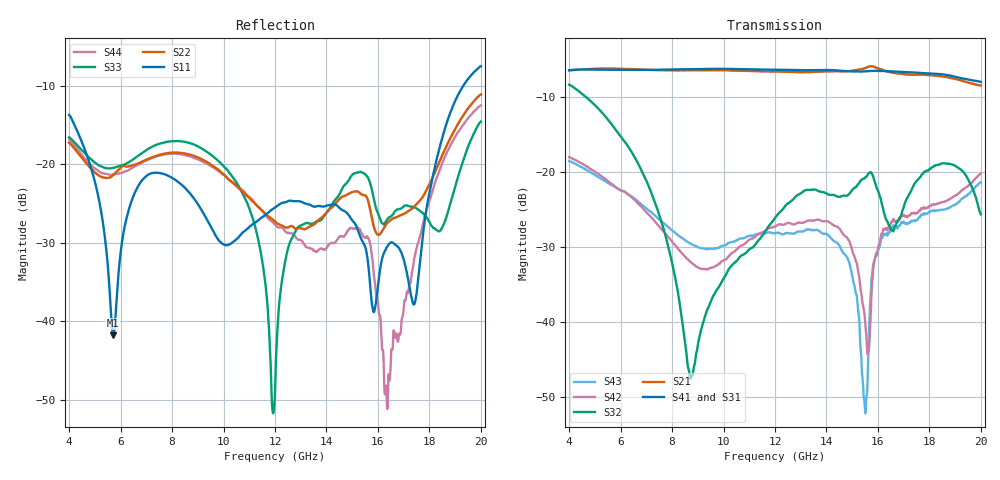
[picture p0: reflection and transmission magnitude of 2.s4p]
!Keysight Technologies,N5247B,US57180241,A.12.85.04
!Date: Friday, March 23, 2018 09:48:32
!Correction: S11(Full 4 Port(1,2,3,4))
!S12(Full 4 Port(1,2,3,4))
!S13(Full 4 Port(1,2,3,4))
!S14(Full 4 Port(1,2,3,4))
!S21(Full 4 Port(1,2,3,4))
!S22(Full 4 Port(1,2,3,4))
!S23(Full 4 Port(1,2,3,4))
!S24(Full 4 Port(1,2,3,4))
!S31(Full 4 Port(1,2,3,4))
!S32(Full 4 Port(1,2,3,4))
!S33(Full 4 Port(1,2,3,4))
!S34(Full 4 Port(1,2,3,4))
!S41(Full 4 Port(1,2,3,4))
!S42(Full 4 Port(1,2,3,4))
!S43(Full 4 Port(1,2,3,4))
!S44(Full 4 Port(1,2,3,4))
!S4P File: Measurements: <S11,S12,S13,S14>,
!<S21,S22,S23,S24>,
!<S31,S32,S33,S34>,
!<S41,S42,S43,S44>:
# Hz S  dB  R 50
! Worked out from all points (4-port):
!   6401 points, 4 GHz to 20 GHz, reference 50 ohm
!   strongest paths, dB at 4 GHz, 8 GHz, 12 GHz, 16 GHz, 20 GHz:
!     S41: -6.4, -6.3, -6.3, -6.5, -8.0
!     S31: -6.5, -6.3, -6.4, -6.6, -7.8
!     S21: -6.4, -6.4, -6.6, -6.2, -8.5
!     S32: -8.3, -32.1, -26.2, -22.5, -25.7
!     S42: -18.0, -29.3, -27.3, -30.3, -20.2
!     S43: -18.5, -27.8, -28.2, -30.6, -21.4
!   lowest |S11| = -41.8 dB at 5.718 GHz (marker M1), VSWR 1.02, Z = 50.6 + j0.581 ohm
!   |S11| at or under -10 dB: start of sweep to 19.31 GHz
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4e9  -13.70 26.3  -6.46 -147.4  -6.54 -148.8  -6.41 -148.1
     -6.42 -147.3  -17.24 -20.4  -8.35 -122.1  -17.99 120.0
     -6.49 -148.8  -8.34 -122.2  -16.55 -25.3  -18.48 118.9
     -6.41 -148.2  -18.03 119.7  -18.54 118.8  -16.80 -23.3
5.7175e9  -41.79 44.8  -6.21 142.2  -6.27 140.9  -6.32 141.8
          -6.20 142.3  -21.36 -29.2  -13.94 -177.9  -21.71 21.9
          -6.26 140.9  -13.94 -178.0  -20.45 -42.5  -21.82 17.1
          -6.35 141.8  -21.75 21.7  -21.86 16.9  -21.27 -38.0
8.74e9  -23.87 -29.6  -6.47 16.7  -6.37 16.2  -6.23 17.7
        -6.42 16.7  -18.81 -104.6  -47.29 9.1  -31.99 160.8
        -6.29 15.8  -47.27 8.7  -17.35 -100.1  -29.47 159.8
        -6.26 17.7  -32.06 160.8  -29.59 160.2  -19.06 -109.5
1.19325e10  -25.65 71.3  -6.52 -122.8  -6.40 -123.4  -6.28 -121.8
            -6.58 -122.8  -27.10 121.9  -26.49 -73.9  -27.36 -107.4
            -6.43 -123.7  -26.46 -74.2  -51.70 79.8  -28.14 -89.6
            -6.35 -121.6  -27.36 -107.2  -28.18 -89.1  -27.45 101.1
1.55075e10  -30.55 -57.7  -6.05 68.9  -6.58 67.5  -6.50 68.1
            -6.11 69.6  -23.97 -53.8  -20.77 -141.2  -40.24 25.6
            -6.59 68.1  -20.71 -141.2  -21.26 -82.7  -52.24 -32.4
            -6.57 69.4  -40.22 26.0  -52.19 -31.8  -29.30 -85.2
1.63225e10  -30.67 61.9  -6.51 22.4  -6.86 26.4  -6.67 27.3
            -6.55 22.1  -27.63 -63.3  -26.68 -170.0  -27.63 43.4
            -6.60 25.6  -26.38 -170.4  -27.25 -74.4  -28.04 56.2
            -6.55 27.2  -27.48 43.5  -28.19 56.8  -48.28 41.1
2e10  -7.50 60.2  -8.18 179.5  -7.91 -174.4  -8.00 -172.5
      -8.46 179.1  -11.10 66.6  -25.99 152.3  -20.56 157.9
      -7.83 -176.9  -25.66 150.1  -14.54 50.6  -21.34 158.0
      -7.96 -174.5  -20.20 156.3  -21.36 158.4  -12.49 55.4
